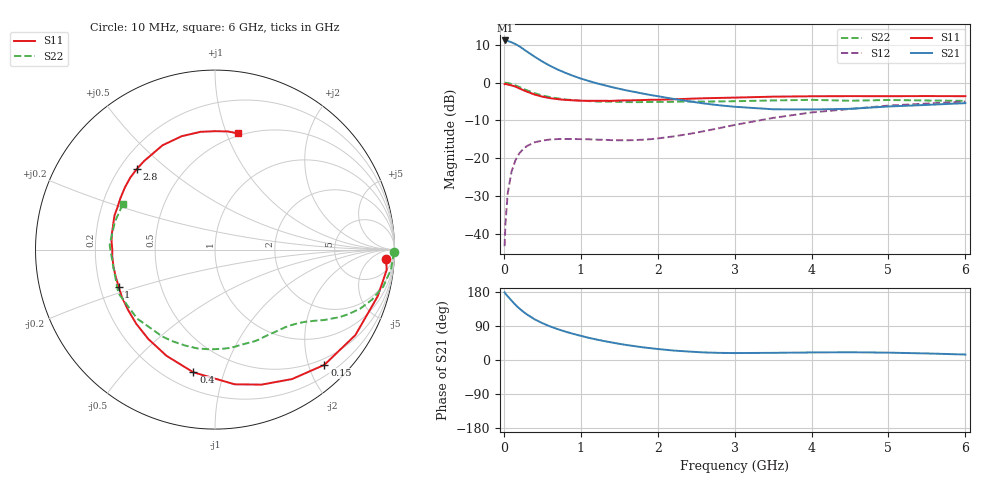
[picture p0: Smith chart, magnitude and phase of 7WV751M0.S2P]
! Infineon Technologies  Discrete & RF Semiconductors
! BFS17W
! Si NPN RF Bipolar Junction Transistor in SOT323
! VCE = 0.75 V  IC = 1 mA
! Common Emitter S-Parameters:  August  1999
# GHz  S  MA  R  50
!  f  S11  S21  S12  S22
! GHz  MAG  ANG  MAG  ANG  MAG  ANG  MAG  ANG
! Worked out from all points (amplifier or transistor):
!   36 points, 10 MHz to 6 GHz, reference 50 ohm
!   highest |S21| = 11.2 dB at 20 MHz (marker M1)
!   |S21| within 3 dB of that: start of sweep to 304.4 MHz
!   unconditionally stable (mu >= 1): 928 MHz to end of sweep
!   at 250 MHz: K = 0.30, MSG = 13.3 dB, |S12| = -17.6 dB
!   at 1.4 GHz: K = 1.39, MAG = 3.3 dB, |S12| = -15.3 dB
!   at 6 GHz: K = 1.14, MAG = -2.5 dB, |S12| = -5.0 dB
!   S11 on the Smith chart (normalised r, x): 10 MHz: 18, -21; 150 MHz: 0.38, -2.27; 400 MHz: 0.30, -0.79; 1 GHz: 0.28, -0.17; 2.8 GHz: 0.27, +0.40; 6 GHz: 0.48, +1.10
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0.01  0.9542 -3.1  3.588 178.4  0.0068 87.7  0.9991 -0.8
0.02  0.9634 -6.7  3.614 175.4  0.0131 85.4  0.9928 -2.6
0.05  0.9431 -16.0  3.56 168.0  0.0339 81.2  0.987 -6.4
0.1  0.9158 -31.3  3.414 156.8  0.066 71.9  0.9598 -12.4
0.15  0.8853 -46.5  3.238 145.8  0.0928 62.7  0.918 -17.7
0.2  0.8395 -59.2  3.03 136.3  0.1151 56.2  0.8749 -22.0
0.25  0.7956 -71.0  2.796 127.8  0.1311 49.3  0.8286 -25.6
0.3  0.7584 -81.7  2.576 120.3  0.1442 44.9  0.7905 -28.4
0.4  0.6943 -100.0  2.204 107.4  0.1616 36.8  0.7226 -32.9
0.5  0.6506 -114.5  1.901 97.4  0.1704 31.3  0.6758 -36.0
0.6  0.6215 -126.7  1.668 88.7  0.176 27.7  0.6414 -38.9
0.8  0.5895 -145.3  1.346 74.9  0.179 23.2  0.598 -44.7
1  0.5755 -158.9  1.131 63.9  0.1781 21.8  0.5767 -50.2
1.1  0.5733 -165.4  1.052 58.7  0.1772 21.7  0.5684 -53.6
1.6  0.5816 171.4  0.785 39.4  0.1719 27.0  0.5516 -70.7
2.2  0.5997 151.4  0.609 25.1  0.1932 40.0  0.5565 -92.5
2.8  0.6259 134.0  0.5 18.8  0.249 47.3  0.5624 -114.4
3.5  0.6506 116.7  0.443 18.9  0.3404 46.2  0.5795 -138.4
4  0.6585 106.4  0.44 19.9  0.402 41.3  0.5906 -155.7
4.5  0.6611 97.0  0.449 20.5  0.4467 35.8  0.5748 -170.7
5.5  0.6623 83.7  0.506 17.3  0.5279 25.2  0.5789 164.6
6  0.6599 78.6  0.534 14.4  0.5606 20.0  0.5728 153.9
